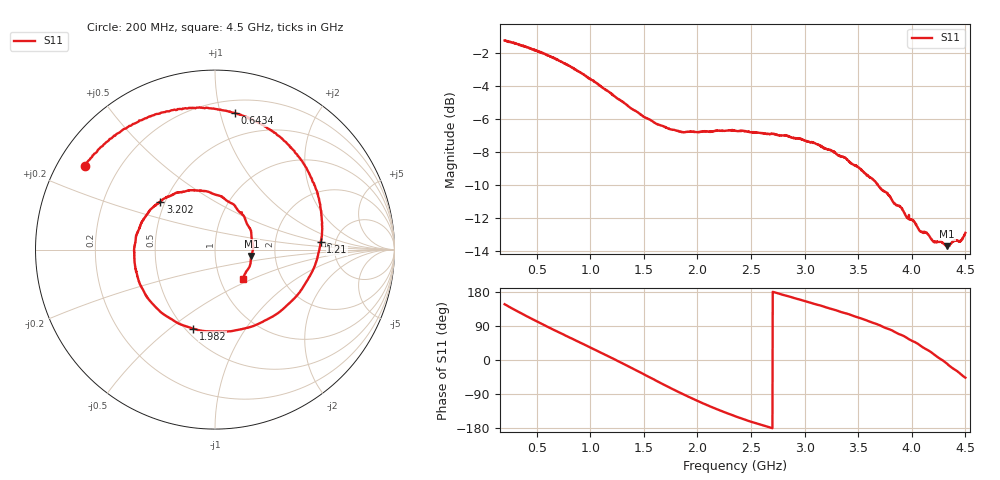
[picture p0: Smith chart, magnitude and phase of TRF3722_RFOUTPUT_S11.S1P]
!Agilent Technologies,E5071B,JP1KK00322,A.09.10
!Date: Thu Dec 19 12:25:43 2013
!Data & Calibration Information:
!Freq	S11:SOLT1(ON)
# Hz S dB R 50
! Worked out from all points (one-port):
!   1601 points, 200 MHz to 4.5 GHz, reference 50 ohm
!   lowest |S11| = -13.7 dB at 4.328 GHz (marker M1), VSWR 1.52, Z = 75.2 - j5.51 ohm
!   |S11| at or under -10 dB: 3.68 GHz to end of sweep
!   S11 on the Smith chart (normalised r, x): 200 MHz: 0.08, +0.29; 643.4 MHz: 0.30, +1.11; 1.21 GHz: 3.82, +0.48; 1.982 GHz: 0.55, -0.61; 3.202 GHz: 0.47, +0.30; 4.5 GHz: 1.28, -0.44
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2e8  -1.27 147.2
3.101875e8  -1.47 129.9
4.176875e8  -1.68 114.0
5.27875e8  -1.99 97.9
6.434375e8  -2.29 81.6
7.375e8  -2.58 68.9
8.61125e8  -3.02 51.9
9.820625e8  -3.55 35.5
1.089562e9  -4.01 20.8
1.2105e9  -4.57 4.0
1.275e9  -4.86 -5.5
1.41475e9  -5.52 -25.3
1.546438e9  -6.04 -44.6
1.678125e9  -6.46 -63.9
1.8125e9  -6.73 -83.0
1.981812e9  -6.81 -105.4
2.169938e9  -6.75 -128.5
2.35e9  -6.73 -148.1
2.591875e9  -6.86 -171.0
2.8875e9  -7.16 164.8
3.201938e9  -7.84 138.7
3.425e9  -8.68 119.7
3.6615e9  -9.84 95.8
3.787812e9  -10.65 81.2
3.9625e9  -12.04 56.9
4.137188e9  -12.89 27.7
4.328e9  -13.72 -9.8
4.5e9  -12.91 -46.6
